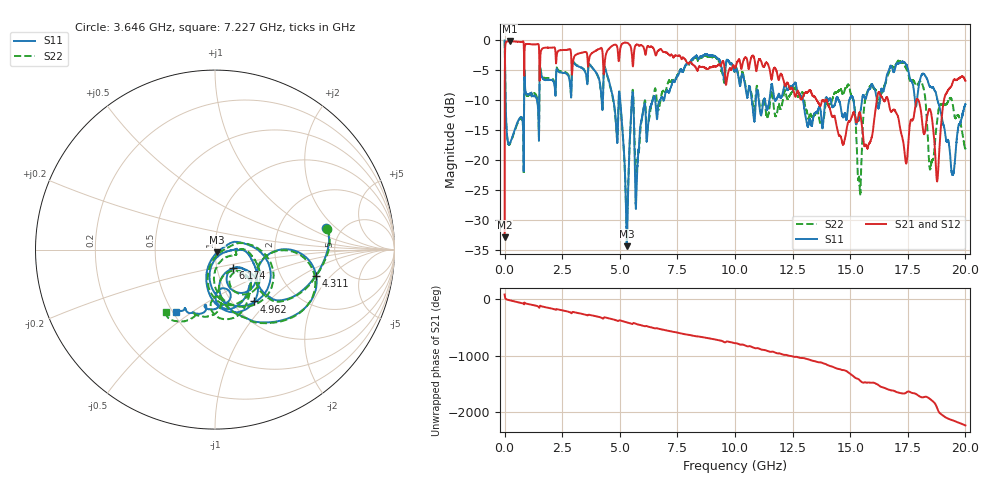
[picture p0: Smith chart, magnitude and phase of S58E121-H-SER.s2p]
!{S58E121}
!Johanson Technology Inc.
!www.johansontechnology.com
!Test Board Conditions:
!Substrate Type  RO4350B
!Substrate Thickness  60 mil
!Substrate Dk  3.66
!TL Type: GCPW
!TL Trace Width  115 mil
!TL Gap  52 mil
!Electrode orientation  Horizontal
!DUT TOPOLOGY	SERIES
!Mounting Pad LxW  55x428 mil
! Created Wed Apr 14 11:06:23 2021
# mhz S ma R 50
! 2 Port Network Data from SP1.SP block
! freq  magS11  angS11  magS21  angS21  magS12  angS12  magS22  angS22
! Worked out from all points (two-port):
!   20001 points, 300 kHz to 20 GHz, reference 50 ohm
!   highest |S21| = -0.14 dB at 218.3 MHz (marker M1); lowest = -32.9 dB at 300 kHz (marker M2)
!   |S21| within 3 dB of the highest: 13.18 MHz to 846.3 MHz (833.1 MHz wide, 194 % of centre); 5.597 GHz to 7.687 GHz (2.09 GHz wide, 31.5 % of centre)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
!   lowest |S11| = -34.4 dB at 5.307 GHz (marker M3), VSWR 1.04, Z = 51.2 - j1.47 ohm
!   |S11| at or under -10 dB: 5.587 GHz to 6.43 GHz (843.2 MHz wide, 14 % of centre); 12.96 GHz to 13.92 GHz (965.5 MHz wide, 7.18 % of centre); 18.79 GHz to end of sweep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
!   |S22| runs from -30.5 to 0.0 dB; largest |S21 - S12| = 0.009
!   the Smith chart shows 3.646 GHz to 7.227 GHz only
!   S11 on the Smith chart (normalised r, x): 3.646 GHz: 3.77, +1.54; 4.311 GHz: 3.13, -1.37; 4.962 GHz: 1.25, -0.83; 6.174 GHz: 1.19, -0.25; 7.227 GHz: 0.52, -0.44
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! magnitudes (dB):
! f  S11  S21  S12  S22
! 300 kHz  0.0  -32.9  -33.0  0.0
! 102.3 MHz  -15.7  -0.2  -0.2  -15.8
! 218.3 MHz  -17.2  -0.1  -0.2  -17.4
! 3.334 GHz  -4.6  -2.1  -2.1  -4.5
! 3.646 GHz  -4.0  -3.8  -3.8  -3.9
! 4.311 GHz  -4.7  -5.5  -5.5  -4.8
! 4.962 GHz  -8.8  -3.4  -3.4  -9.9
! 5.307 GHz  -34.4  -0.4  -0.4  -30.4
! 5.521 GHz  -10.2  -2.1  -2.1  -10.0
! 5.735 GHz  -23.8  -0.7  -0.7  -21.7
! 6.174 GHz  -16.8  -1.2  -1.2  -15.6
! 6.667 GHz  -10.8  -1.7  -1.8  -11.6
! 7.227 GHz  -7.7  -2.4  -2.4  -7.1
! 10 GHz  -5.1  -4.6  -4.6  -5.0
! 13.33 GHz  -14.3  -9.0  -9.0  -12.8
! 14.92 GHz  -10.7  -13.6  -13.7  -7.4
! 15.4 GHz  -13.0  -12.0  -12.1  -23.5
! 15.72 GHz  -9.1  -17.9  -17.8  -8.8
! 16.67 GHz  -5.1  -10.4  -10.5  -5.5
! 18.78 GHz  -9.8  -23.6  -23.6  -13.3
! 19.45 GHz  -22.5  -7.0  -7.0  -10.6
! 20 GHz  -10.6  -6.8  -6.8  -18.0
